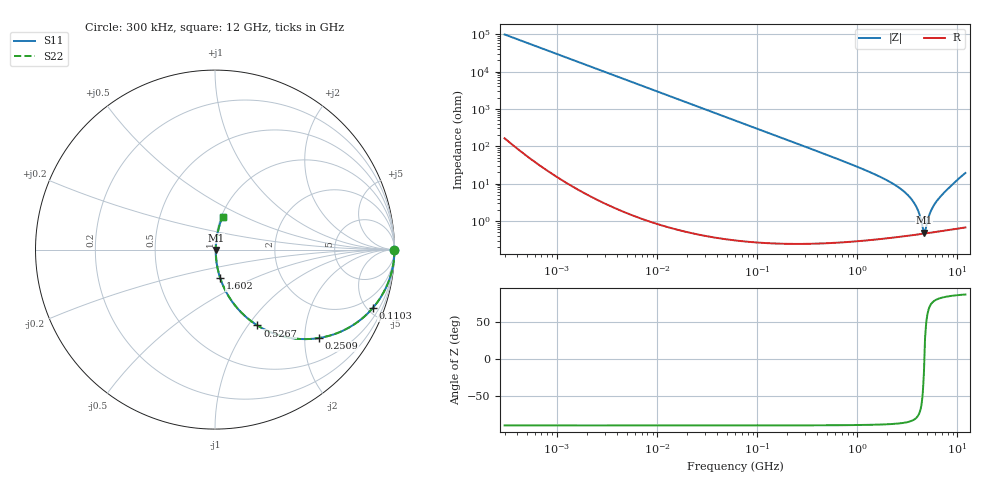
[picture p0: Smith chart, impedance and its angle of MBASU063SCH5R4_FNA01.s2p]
! MBASU063SCH5R4_FNA01  S-PARAMETER MODEL  ( General Type )
! Model Generated by TAIYO YUDEN Corporation (http://www.ty-top.com)
! Version 1.0
! TAIYO YUDEN Control No. 130801
! Copyright(c) 2013 TAIYO YUDEN CO.,LTD. All Rights Reserved.
! Product Description (link to TY-COMPAS)
! https://ds.yuden.co.jp/TYCOMPAS/or/detail?pn=MBASU063SCH5R4DFNA01&u=M
! Products Name : Multilayer Ceramic Capacitors
! Characteristics :
!  Capacitance : 5.4 pF , Rated Voltage : 50V , TCC : CH / C0H
!  Case Size : 0.6 x 0.3 / 0.024 x 0.012 [mm/inch] , Thickness : 0.3 / 0.012 [mm/inch]
!  (Conditions: Temperature = 25 degC , DC Bias Current/Voltage = 0A / 0V)
! External Node Assignments :
!  1  o---| |---o  2
! GND o---------o GND
! Frequency Range : 0.3MHz  -  12000MHz  [ 401 STEP ]
# MHz S RI R 50
! Freq[MHz].  S11 Real  S11 Imag  S21 Real  S21 Imag  S12 Real  S12 Imag  S22 Real  S22 Imag
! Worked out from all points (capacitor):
!   401 points, 300 kHz to 12 GHz, reference 50 ohm
!   read as one part in series: C = 5.37 pF near 316.3 kHz
!   lowest |Z| = 484 mohm at 4.624 GHz (marker M1)
!   series resonance near 4.67 GHz, so ESL is about 220 pH
!   S11 on the Smith chart (normalised r, x): 300 kHz: open; 110.3 MHz: 1.01, -5.36; 250.9 MHz: 1.00, -2.35; 526.7 MHz: 1.01, -1.11; 1.602 GHz: 1.01, -0.33; 12 GHz: 1.01, +0.39
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0.3  1 -0.00101  2.71e-06 0.00101  2.71e-06 0.00101  1 -0.00101
1.769972  1 -0.00598  3.79e-05 0.00598  3.79e-05 0.00598  1 -0.00598
10.44266  0.9987 -0.0352  0.00125 0.0352  0.00125 0.0352  0.9987 -0.0352
60  0.9604 -0.1946  0.0396 0.1946  0.0396 0.1946  0.9604 -0.1946
110.3493  0.8777 -0.3271  0.1223 0.3271  0.1223 0.3271  0.8777 -0.3271
250.8588  0.5806 -0.4924  0.4194 0.4924  0.4194 0.4924  0.5806 -0.4924
353.9943  0.4092 -0.4902  0.5908 0.4902  0.5908 0.4902  0.4092 -0.4902
526.7124  0.2366 -0.4227  0.7634 0.4227  0.7634 0.4227  0.2366 -0.4227
871.3074  0.0992 -0.2947  0.9008 0.2947  0.9008 0.2947  0.0992 -0.2947
1602.47  0.0289 -0.1579  0.9711 0.1579  0.9711 0.1579  0.0289 -0.1579
2088.533  0.0161 -0.1113  0.9839 0.1113  0.9839 0.1113  0.0161 -0.1113
2870.14  0.00793 -0.0635  0.9921 0.0635  0.9921 0.0635  0.00793 -0.0635
3547.679  0.00539 -0.0351  0.9946 0.0351  0.9946 0.0351  0.00539 -0.0351
3944.255  0.00478 -0.0214  0.9952 0.0214  0.9952 0.0214  0.00478 -0.0214
4502.883  0.00455 -0.0047  0.9954 0.0047  0.9954 0.0047  0.00455 -0.0047
4623.766  0.00458 -0.00152  0.9954 0.00152  0.9954 0.00152  0.00458 -0.00152
4875.354  0.0047 0.00552  0.9953 -0.00552  0.9953 -0.00552  0.0047 0.00552
5278.635  0.00502 0.0146  0.995 -0.0146  0.995 -0.0146  0.00502 0.0146
5565.855  0.00534 0.0206  0.9947 -0.0206  0.9947 -0.0206  0.00534 0.0206
6354.153  0.00649 0.0363  0.9935 -0.0363  0.9935 -0.0363  0.00649 0.0363
8966.534  0.015 0.0945  0.985 -0.0945  0.985 -0.0945  0.015 0.0945
12000  0.042 0.1839  0.958 -0.1839  0.958 -0.1839  0.042 0.1839
